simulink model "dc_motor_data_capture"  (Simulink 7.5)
settings: Solver=FixedStepDiscrete  StartTime=0.0  StopTime=40  FixedStep=0.001  RelTol=1e-3
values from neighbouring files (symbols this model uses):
  bits = 32    [hexcalc.m]
undefined symbols (not defined in the file or in its folder): bin2dec, Buffer, characters, contain, DiscIntNeverNeededParam, full, is, PWM, Receive, When
libraries: dsPICdrivers x9, simulink x1

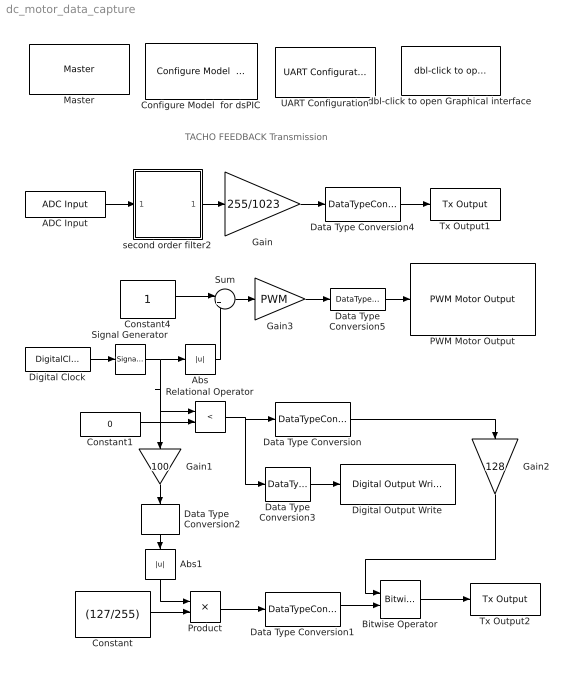
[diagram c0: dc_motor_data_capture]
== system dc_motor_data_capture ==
  note: TACHO FEEDBACK Transmission
  ADC Input : dsPICdrivers/Peripheral I//O/ADC Input  Tag=dsPIC_ADC  Priority=5  ADC_TYPE=10 bits  ADC_MODE=Continuous sampling & get last channel value  NbrSampleStep=1  VoltRefpopup="AVdd  -  AVss"  OutFormatBitspopup=0000 00dd dddd dddd : Integer  InterruptPriority=6  ANCHANNELS=[3]  MaxName=ANmax = 1023  Rin=1e2  ADCS=1  SAMC=1  Temperature=25  DMAChannel=0  SampleTime=0.001  Status="OK  |  Tsmp=1.600e-007 |  T/Channel=2.080e-006 |  Tall=2.080e-006"  SSRC=auto convert
  Abs : Abs  OutDataType=fixdt(1, 16)  OutScaling=2^0
  Abs1 : Abs  OutDataType=fixdt(1, 16)  OutScaling=2^0
  Bitwise Operator : simulink/Logic and Bit Operations/Bitwise Operator  logicop=OR  UseBitMask=off  NumInputPorts=2  BitMask=bin2dec('11011001')  BitMaskRealWorld=Stored Integer
  Configure Model  for dsPIC : dsPICdrivers/Simulink Configuration/Configure Model  for dsPIC
  Constant : Constant  Value=(127/255)  OutDataTypeMode=Specify via dialog  OutDataType=fixdt(1,16)  ConRadixGroup=Best Precision: Vector-wise  OutDataTypeStr=fixdt(1,16)
  Constant1 : Constant  Value=0  OutDataType=fixdt(1, 16)  OutScaling=2^0
  Constant4 : Constant  OutDataType=fixdt(1, 16)  OutScaling=2^0
  Data Type Conversion : DataTypeConversion  OutDataTypeMode=uint8  OutDataType=fixdt(1, 16)  OutScaling=2^0  OutDataTypeStr=uint8
  Data Type Conversion1 : DataTypeConversion  OutDataTypeMode=uint8  OutDataType=fixdt(1, 16)  OutScaling=2^0  OutDataTypeStr=uint8
  Data Type Conversion2 : DataTypeConversion  OutDataTypeMode=int8  OutDataType=fixdt(1, 16)  OutScaling=2^0  OutDataTypeStr=int8
  Data Type Conversion3 : DataTypeConversion  OutDataTypeMode=boolean  OutDataType=fixdt(1, 16)  OutScaling=2^0  OutDataTypeStr=boolean
  Data Type Conversion4 : DataTypeConversion  OutDataTypeMode=uint8  OutDataType=fixdt(1, 16)  OutScaling=2^0  OutDataTypeStr=uint8  RndMeth=Convergent
  Data Type Conversion5 : DataTypeConversion  OutDataTypeMode=uint16  OutDataType=fixdt(1, 16)  OutScaling=2^0  OutDataTypeStr=uint16  SampleTime=0.001
  Digital Clock : DigitalClock  SampleTime=0.001
  Digital Output Write : dsPICdrivers/Digital I//O/Digital Output Write  Tag=dsPIC_Digital_Output  Priority=5  PORT=D  Pin=[1]  Simultaneous=off  OrderingInOutPopup=None
  Gain : Gain  Gain=255/1023  ParameterDataType=fixdt(1, 16)  ParameterScaling=2^0  OutDataType=fixdt(1, 16)  OutScaling=2^0
  Gain1 : Gain  Gain=100  ParameterDataType=fixdt(1, 16)  ParameterScaling=2^0  OutDataTypeMode=int8  OutDataType=fixdt(1, 16)  OutScaling=2^0  OutDataTypeStr=int8
  Gain2 : Gain  Gain=128  ParameterDataType=fixdt(1, 16)  ParameterScaling=2^0  OutDataTypeMode=uint8  OutDataType=fixdt(1, 16)  OutScaling=2^0  OutDataTypeStr=uint8
  Gain3 : Gain  Gain=PWM  ParameterDataType=fixdt(1, 16)  ParameterScaling=2^0  OutDataType=fixdt(1, 16)  OutScaling=2^0  SampleTime=0.001
  Master : dsPICdrivers/Master  Tag=dsPIC_MASTER  Priority=1  TimeStepType=Timer1  picType=30f4012  fcy=6.25e6  Quartz_33f=5e6  PLLActive_33f=off  fcyDesired_33f=0  tmr1="[1  6249  0]"  tmr1Info="Time Step : 0.001  ;   Error : 0%  PR1=6249"  tmr2345="[0  0  0  0]"  tmr2345cfg=[-1 -1 -1 -1]  IOautoConf=on  typePort="[ 0   0   0   0   0   0   0   0   0   0   0   0   0   0   0   0   0   0   0   8   0   0   0   0   0   0   0   0   0   0   0   0   0   0   0   0   0   0   0   0   0   0   0   0   0   0   0   0   0  10   0   0   0   0   0   0   0   0   0   0   0   0   0   0   0   0   0   0   0   0   0   0   0   0   0   0   0   0   0   0   0   0   4   5   0   0   0   0   0   0   0   0   0   0   0   0   0   0   0   0 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"  TRIS="[ 65535  65535  65535  65533  65535  65535  65535 ]"  ADPCFG=0  MasterBusyPort=None  MasterOverloadPort=None  FOSC=HS  ClockSwitchMonitor=Both disabled  TempProtection_33f=TEMP_ON  FPBOR=PBOR_OFF  PWRT=PWRT_OFF  MCLR=MCLR_DIS  ICD=ICS_NONE  JTAGEN=JTAGEN_OFF  PowerSave=off  OverrideFcy=off  NewFcy=1e6  PR2345="[65535  65535  65535  65535]"
  PWM Motor Output : dsPICdrivers/Peripheral I//O/PWM Motor Output  Tag=dsPIC_PWM_Motor  Priority=5  PWMref=1  PWM12=1  InputEnableChk=off  InputPeriodeChk=off  Channel=[1]  TPeriode=10e-3  PrescalerValue=4  PeriodeInteger=15625  MaxName='PWM'  Centered=off  HChannelON=off  Info="Nbr Bits : 14.9316  ||  PWM = 31250  ||  Prescaler = 4"  Delay=0  IntPriority=5  nbrPwmChannelPIC=3  Status=OK  DeadTimePrescaleA=0  DeadTimePrescaleB=0  DeadTimeInfo=Dead Time A = 0  DTPWM1a=Prescaler A  DTPWM1i=Prescaler A  DTPWM2a=Prescaler A  DTPWM2i=Prescaler A  DTPWM3a=Prescaler A  DTPWM3i=Prescaler A  DTPWM4a=Prescaler A  DTPWM4i=Prescaler A  DTCON1=0  DTCON2=0
  Product : Product
  Relational Operator : RelationalOperator  Operator=<  LogicOutDataTypeMode=boolean  LogicDataType=fixdt(0, 8)  OutDataTypeStr=boolean
  Signal Generator : SignalGenerator  WaveForm=square  TimeSource=Use external signal  Amplitude=(1-0.4)  Frequency=1/10
  Sum : Sum  Inputs=|+-  OutDataType=fixdt(1, 16)  OutScaling=2^0
  Tx Output1 : dsPICdrivers/Serial PORT/Tx Output  Tag=dsPIC_TX  Priority=5  UART=1  OrderingInOutPopup=None
  Tx Output2 : dsPICdrivers/Serial PORT/Tx Output  Tag=dsPIC_TX  Priority=5  UART=1  OrderingInOutPopup=None
  UART Configuration : dsPICdrivers/Serial PORT/UART Configuration  Tag=dsPIC_config_UART  Priority=2  UART=1  proposed_BAUD=57600  ALT_TX_RX=off  InterruptTxWhen=When Transmit Buffer is empty  TXInterruptPri=1  TxBufferSize=32  TXEN=on  InterruptRxWhen=When Receive Buffer is full (contain 4 characters)  RXInterruptPri=2  RxBufferSize=32  BAUD=57600  UxBRG=6  Info="UxBRG = 6   ||  Real Baud : 55804   ||  % error : -3.1188  ||  max 5.5804 Bytes / Step"  RealBaud=0
  dbl-click to open Graphical interface : dsPICdrivers/Serial PORT/dbl-click to open Graphical interface  Nothing=0
  second order filter2 : Subsystem
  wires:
  Data Type Conversion3/1 -> Digital Output Write/1
  Data Type Conversion/1 -> Gain2/1
  Constant4/1 -> Sum/1
  Abs/1 -> Sum/2
  Sum/1 -> Gain3/1
  Data Type Conversion5/1 -> PWM Motor Output/1
  Gain3/1 -> Data Type Conversion5/1
  Digital Clock/1 -> Signal Generator/1
  Constant1/1 -> Relational Operator/2
  Relational Operator/1 -> Data Type Conversion/1, Data Type Conversion3/1
  Bitwise Operator/1 -> Tx Output2/1
  Gain2/1 -> Bitwise Operator/1
  Product/1 -> Data Type Conversion1/1
  Constant/1 -> Product/2
  Data Type Conversion1/1 -> Bitwise Operator/2
  Data Type Conversion2/1 -> Abs1/1
  Gain1/1 -> Data Type Conversion2/1
  Abs1/1 -> Product/1
  Data Type Conversion4/1 -> Tx Output1/1
  Gain/1 -> Data Type Conversion4/1
  ADC Input/1 -> second order filter2/1(In1)
  second order filter2/1(Out1) -> Gain/1
  Signal Generator/1 -> Abs/1, Relational Operator/1, Gain1/1

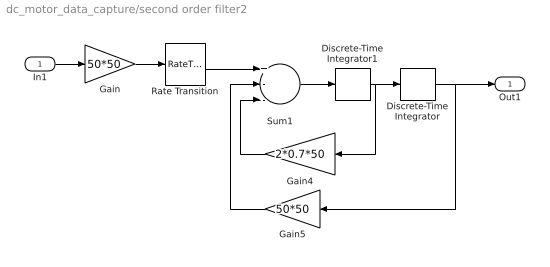
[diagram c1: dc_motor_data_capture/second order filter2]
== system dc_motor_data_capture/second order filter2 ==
  In1 : Inport  OutDataType=fixdt(1, 16)  OutScaling=2^0
  Discrete-Time Integrator : DiscreteIntegrator  SampleTime=0.001  OutDataTypeMode=double  OutDataType=fixdt(1, 16)  OutScaling=2^0  OutDataTypeStr=double  ICPrevOutput=DiscIntNeverNeededParam  ICPrevScaledInput=DiscIntNeverNeededParam
  Discrete-Time Integrator1 : DiscreteIntegrator  SampleTime=0.001  OutDataTypeMode=double  OutDataType=fixdt(1, 16)  OutScaling=2^0  OutDataTypeStr=double  ICPrevOutput=DiscIntNeverNeededParam  ICPrevScaledInput=DiscIntNeverNeededParam
  Gain : Gain  Gain=50*50  ParameterDataType=fixdt(1, 16)  ParameterScaling=2^0  OutDataTypeMode=double  OutDataType=fixdt(1, 16)  OutScaling=2^0  OutDataTypeStr=double
  Gain4 : Gain  Gain=2*0.7*50  ParameterDataType=fixdt(1, 16)  ParameterScaling=2^0  OutDataTypeMode=double  OutDataType=fixdt(1, 16)  OutScaling=2^0  OutDataTypeStr=double
  Gain5 : Gain  Gain=50*50  ParameterDataType=fixdt(1, 16)  ParameterScaling=2^0  OutDataTypeMode=double  OutDataType=fixdt(1, 16)  OutScaling=2^0  OutDataTypeStr=double
  Rate Transition : RateTransition  Integrity=off  Deterministic=off  OutPortSampleTime=0.001
  Sum1 : Sum  Inputs=+--  OutDataTypeMode=double  OutDataType=fixdt(1, 16)  OutScaling=2^0  OutDataTypeStr=double  SampleTime=0.001
  Out1 : Outport  OutDataType=fixdt(1, 16)  OutScaling=2^0
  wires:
  Rate Transition/1 -> Sum1/1
  In1/1 -> Gain/1
  Gain5/1 -> Sum1/2
  Discrete-Time Integrator/1 -> Out1/1, Gain5/1
  Gain4/1 -> Sum1/3
  Sum1/1 -> Discrete-Time Integrator1/1
  Discrete-Time Integrator1/1 -> Discrete-Time Integrator/1, Gain4/1
  Gain/1 -> Rate Transition/1
